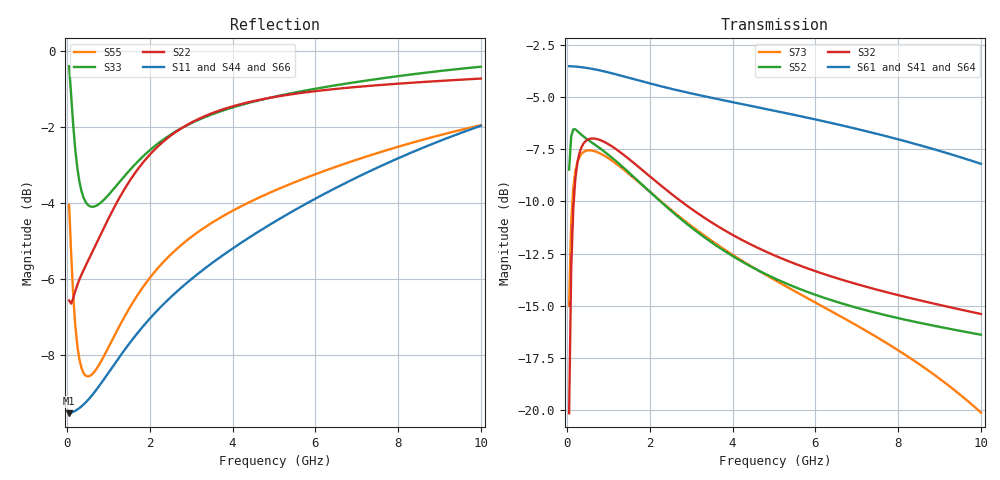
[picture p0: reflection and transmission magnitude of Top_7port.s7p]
! Created Mon Dec 14 12:31:43 2020
# ghz S ma R 50
! 7 Port Network Data from SP1.SP block
! freq  magS11  angS11  magS12  angS12  magS13  angS13  magS14  angS14
!  magS15  angS15  magS16  angS16  magS17  angS17
!  magS21  angS21
!  magS22  angS22  magS23  angS23  magS24  angS24  magS25  angS25
!  magS26  angS26  magS27  angS27
!  magS31  angS31  magS32  angS32
!  magS33  angS33  magS34  angS34  magS35  angS35  magS36  angS36
!  magS37  angS37
!  magS41  angS41  magS42  angS42  magS43  angS43
!  magS44  angS44  magS45  angS45  magS46  angS46  magS47  angS47
!  magS51  angS51  magS52  angS52  magS53  angS53  magS54  angS54
!  magS55  angS55  magS56  angS56  magS57  angS57
!  magS61  angS61
!  magS62  angS62  magS63  angS63  magS64  angS64  magS65  angS65
!  magS66  angS66  magS67  angS67
!  magS71  angS71  magS72  angS72
!  magS73  angS73  magS74  angS74  magS75  angS75  magS76  angS76
!  magS77  angS77
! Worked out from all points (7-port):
!   200 points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, 50 MHz to 10 GHz, reference 50 ohm
!   strongest paths, dB at 50 MHz, 2.55 GHz, 5.05 GHz, 7.55 GHz, 10 GHz:
!     S61: -3.5, -4.6, -5.7, -6.8, -8.2
!     S41: -3.5, -4.6, -5.7, -6.8, -8.2
!     S64: -3.5, -4.6, -5.7, -6.8, -8.3
!     S32: -20.1, -9.7, -12.6, -14.3, -15.4
!     S52: -8.5, -10.5, -13.7, -15.4, -16.4
!     S73: -15.0, -10.5, -13.8, -16.6, -20.1
!   lowest |S11| = -9.5 dB at 50 MHz (marker M1), VSWR 2.00, Z = 25 - j0.325 ohm
!   |S11| at or under -10 dB: nowhere
